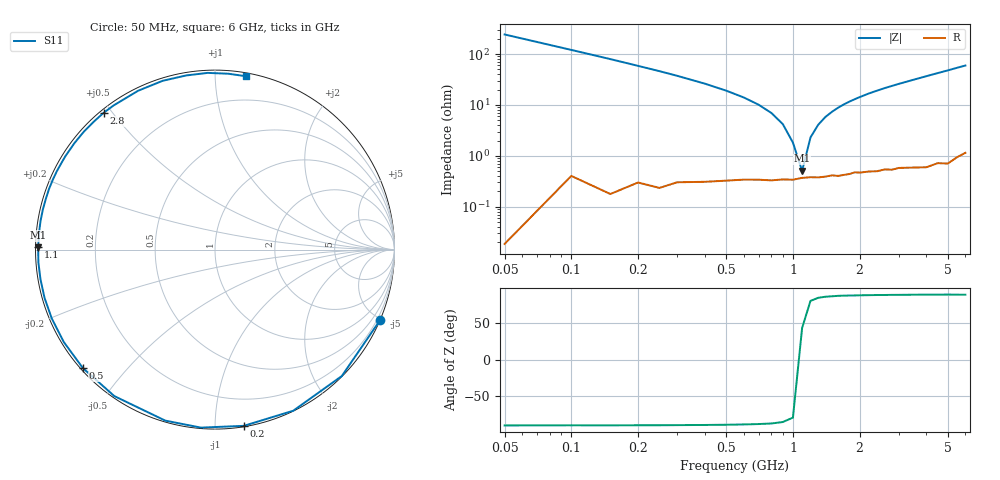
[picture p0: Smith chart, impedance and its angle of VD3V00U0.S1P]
! Infineon Technologies  Discrete & RF Semiconductors
! BBY 55-03
! Si Tuning Diode in SOD323
! VR = 3 V
! S-Parameters:  June  1999
# GHz  S  MA  R  50
!  f  S11
! GHz  MAG  ANG
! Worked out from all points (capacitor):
!   34 points, 50 MHz to 6 GHz, reference 50 ohm
!   read as one part to ground: C = 13 pF near 50 MHz
!   lowest |Z| = 508 mohm at 1.1 GHz (marker M1)
!   series resonance near 1.084 GHz, so ESL is about 1.7 nH
!   S11 on the Smith chart (normalised r, x): 50 MHz: 0.00, -4.87; 200 MHz: 0.01, -1.18; 500 MHz: 0.01, -0.38; 1.1 GHz: 0.01, +0.01; 2.8 GHz: 0.01, +0.47; 6 GHz: 0.02, +1.19
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0.05  1 -23.2
0.1  0.9977 -44.9
0.15  0.998 -64.1
0.2  0.995 -80.7
0.25  0.995 -94.5
0.3  0.9923 -106.2
0.4  0.9904 -124.5
0.5  0.9887 -138.1
0.6  0.9874 -148.6
0.7  0.987 -157.1
0.8  0.9871 -164.2
0.9  0.9864 -170.4
1.1  0.9853 179.2
1.2  0.9849 174.8
1.4  0.9847 166.8
1.6  0.9845 159.9
1.8  0.9835 153.7
2  0.9828 148.1
2.2  0.9825 142.8
2.4  0.9827 138.0
2.8  0.9827 129.2
3  0.9819 125.1
3.5  0.9832 115.8
4  0.9847 107.2
4.5  0.9834 99.4
5  0.9854 92.4
5.5  0.9827 85.7
6  0.9812 79.9
